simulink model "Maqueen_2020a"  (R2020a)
settings: Solver=VariableStepAuto  StartTime=0.0  StopTime=2  RelTol=1e-3
model workspace: external: MAT-File (data not in the file)
undefined symbols (not defined in the file or in its folder): deg, kg, m, mm, N, rad, s, smiData, X, Y, Z
libraries: sm_lib x459, fl_lib x12, nesl_utility x10
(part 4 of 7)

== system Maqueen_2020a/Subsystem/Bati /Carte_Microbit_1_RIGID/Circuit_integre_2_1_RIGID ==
  ReferenceFrame : sm_lib/Frames and Transforms/Reference Frame
  Solid : sm_lib/Body Elements/File Solid  ExtGeomFileName=Circuit integre 2_Defaut_sldprt.STL  UnitType=Custom  ExtGeomFileUnits=mm  StepReaderType=HEX  ExportConvexHullGeometry=off  InertiaType=Custom  Mass=smiData.Solid(13).mass  MassUnits=kg  CenterOfMass=smiData.Solid(13).CoM  CenterOfMassUnits=mm  MomentsOfInertia=smiData.Solid(13).MoI  MomentsOfInertiaUnits=kg*mm^2  ProductsOfInertia=smiData.Solid(13).PoI  ProductsOfInertiaUnits=kg*mm^2  BasedOnType=Density  Density=1000  DensityUnits=kg/m^3  DoExposeReferenceFrame=on  SerializedFrames=<Frames/>  GraphicType=FromGeometry  MarkerShape=Sphere  MarkerSize=10  GraphicVisPropType=SimpleVisualProperties  GraphicDiffuseColor=smiData.Solid(13).color  GraphicSpecularColor=[0.5 0.5 0.5 1.0]  GraphicAmbientColor=[0.15 0.15 0.15 1.0]  GraphicEmissiveColor=[0.0 0.0 0.0 1.0]  GraphicShininess=75  GraphicOpacity=smiData.Solid(13).opacity
  F : PMIOPort  Side=Left
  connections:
  ReferenceFrame/RConn1 -- Solid/RConn1 -- F/RConn1

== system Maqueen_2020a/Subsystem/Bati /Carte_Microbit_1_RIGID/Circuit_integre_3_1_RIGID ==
  ReferenceFrame : sm_lib/Frames and Transforms/Reference Frame
  Solid : sm_lib/Body Elements/File Solid  ExtGeomFileName=Circuit integre 3_Defaut_sldprt.STL  UnitType=Custom  ExtGeomFileUnits=mm  StepReaderType=HEX  ExportConvexHullGeometry=off  InertiaType=Custom  Mass=smiData.Solid(17).mass  MassUnits=kg  CenterOfMass=smiData.Solid(17).CoM  CenterOfMassUnits=mm  MomentsOfInertia=smiData.Solid(17).MoI  MomentsOfInertiaUnits=kg*mm^2  ProductsOfInertia=smiData.Solid(17).PoI  ProductsOfInertiaUnits=kg*mm^2  BasedOnType=Density  Density=1000  DensityUnits=kg/m^3  DoExposeReferenceFrame=on  SerializedFrames=<Frames/>  GraphicType=FromGeometry  MarkerShape=Sphere  MarkerSize=10  GraphicVisPropType=SimpleVisualProperties  GraphicDiffuseColor=smiData.Solid(17).color  GraphicSpecularColor=[0.5 0.5 0.5 1.0]  GraphicAmbientColor=[0.15 0.15 0.15 1.0]  GraphicEmissiveColor=[0.0 0.0 0.0 1.0]  GraphicShininess=75  GraphicOpacity=smiData.Solid(17).opacity
  F : PMIOPort  Side=Left
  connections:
  ReferenceFrame/RConn1 -- Solid/RConn1 -- F/RConn1

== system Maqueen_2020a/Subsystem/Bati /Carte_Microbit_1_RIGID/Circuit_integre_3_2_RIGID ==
  ReferenceFrame : sm_lib/Frames and Transforms/Reference Frame
  Solid : sm_lib/Body Elements/File Solid  ExtGeomFileName=Circuit integre 3_Defaut_sldprt.STL  UnitType=Custom  ExtGeomFileUnits=mm  StepReaderType=HEX  ExportConvexHullGeometry=off  InertiaType=Custom  Mass=smiData.Solid(17).mass  MassUnits=kg  CenterOfMass=smiData.Solid(17).CoM  CenterOfMassUnits=mm  MomentsOfInertia=smiData.Solid(17).MoI  MomentsOfInertiaUnits=kg*mm^2  ProductsOfInertia=smiData.Solid(17).PoI  ProductsOfInertiaUnits=kg*mm^2  BasedOnType=Density  Density=1000  DensityUnits=kg/m^3  DoExposeReferenceFrame=on  SerializedFrames=<Frames/>  GraphicType=FromGeometry  MarkerShape=Sphere  MarkerSize=10  GraphicVisPropType=SimpleVisualProperties  GraphicDiffuseColor=smiData.Solid(17).color  GraphicSpecularColor=[0.5 0.5 0.5 1.0]  GraphicAmbientColor=[0.15 0.15 0.15 1.0]  GraphicEmissiveColor=[0.0 0.0 0.0 1.0]  GraphicShininess=75  GraphicOpacity=smiData.Solid(17).opacity
  F : PMIOPort  Side=Left
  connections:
  ReferenceFrame/RConn1 -- Solid/RConn1 -- F/RConn1

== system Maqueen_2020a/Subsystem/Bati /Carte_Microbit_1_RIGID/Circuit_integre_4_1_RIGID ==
  ReferenceFrame : sm_lib/Frames and Transforms/Reference Frame
  Solid : sm_lib/Body Elements/File Solid  ExtGeomFileName=Circuit integre 4_Defaut_sldprt.STL  UnitType=Custom  ExtGeomFileUnits=mm  StepReaderType=HEX  ExportConvexHullGeometry=off  InertiaType=Custom  Mass=smiData.Solid(12).mass  MassUnits=kg  CenterOfMass=smiData.Solid(12).CoM  CenterOfMassUnits=mm  MomentsOfInertia=smiData.Solid(12).MoI  MomentsOfInertiaUnits=kg*mm^2  ProductsOfInertia=smiData.Solid(12).PoI  ProductsOfInertiaUnits=kg*mm^2  BasedOnType=Density  Density=1000  DensityUnits=kg/m^3  DoExposeReferenceFrame=on  SerializedFrames=<Frames/>  GraphicType=FromGeometry  MarkerShape=Sphere  MarkerSize=10  GraphicVisPropType=SimpleVisualProperties  GraphicDiffuseColor=smiData.Solid(12).color  GraphicSpecularColor=[0.5 0.5 0.5 1.0]  GraphicAmbientColor=[0.15 0.15 0.15 1.0]  GraphicEmissiveColor=[0.0 0.0 0.0 1.0]  GraphicShininess=75  GraphicOpacity=smiData.Solid(12).opacity
  F : PMIOPort  Side=Left
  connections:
  ReferenceFrame/RConn1 -- Solid/RConn1 -- F/RConn1

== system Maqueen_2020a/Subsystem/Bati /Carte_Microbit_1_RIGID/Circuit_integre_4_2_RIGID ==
  ReferenceFrame : sm_lib/Frames and Transforms/Reference Frame
  Solid : sm_lib/Body Elements/File Solid  ExtGeomFileName=Circuit integre 4_Defaut_sldprt.STL  UnitType=Custom  ExtGeomFileUnits=mm  StepReaderType=HEX  ExportConvexHullGeometry=off  InertiaType=Custom  Mass=smiData.Solid(12).mass  MassUnits=kg  CenterOfMass=smiData.Solid(12).CoM  CenterOfMassUnits=mm  MomentsOfInertia=smiData.Solid(12).MoI  MomentsOfInertiaUnits=kg*mm^2  ProductsOfInertia=smiData.Solid(12).PoI  ProductsOfInertiaUnits=kg*mm^2  BasedOnType=Density  Density=1000  DensityUnits=kg/m^3  DoExposeReferenceFrame=on  SerializedFrames=<Frames/>  GraphicType=FromGeometry  MarkerShape=Sphere  MarkerSize=10  GraphicVisPropType=SimpleVisualProperties  GraphicDiffuseColor=smiData.Solid(12).color  GraphicSpecularColor=[0.5 0.5 0.5 1.0]  GraphicAmbientColor=[0.15 0.15 0.15 1.0]  GraphicEmissiveColor=[0.0 0.0 0.0 1.0]  GraphicShininess=75  GraphicOpacity=smiData.Solid(12).opacity
  F : PMIOPort  Side=Left
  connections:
  ReferenceFrame/RConn1 -- Solid/RConn1 -- F/RConn1

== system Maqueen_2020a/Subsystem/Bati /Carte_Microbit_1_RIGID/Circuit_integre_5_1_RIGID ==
  ReferenceFrame : sm_lib/Frames and Transforms/Reference Frame
  Solid : sm_lib/Body Elements/File Solid  ExtGeomFileName=Circuit integre 5_Defaut_sldprt.STL  UnitType=Custom  ExtGeomFileUnits=mm  StepReaderType=HEX  ExportConvexHullGeometry=off  InertiaType=Custom  Mass=smiData.Solid(14).mass  MassUnits=kg  CenterOfMass=smiData.Solid(14).CoM  CenterOfMassUnits=mm  MomentsOfInertia=smiData.Solid(14).MoI  MomentsOfInertiaUnits=kg*mm^2  ProductsOfInertia=smiData.Solid(14).PoI  ProductsOfInertiaUnits=kg*mm^2  BasedOnType=Density  Density=1000  DensityUnits=kg/m^3  DoExposeReferenceFrame=on  SerializedFrames=<Frames/>  GraphicType=FromGeometry  MarkerShape=Sphere  MarkerSize=10  GraphicVisPropType=SimpleVisualProperties  GraphicDiffuseColor=smiData.Solid(14).color  GraphicSpecularColor=[0.5 0.5 0.5 1.0]  GraphicAmbientColor=[0.15 0.15 0.15 1.0]  GraphicEmissiveColor=[0.0 0.0 0.0 1.0]  GraphicShininess=75  GraphicOpacity=smiData.Solid(14).opacity
  F : PMIOPort  Side=Left
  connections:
  ReferenceFrame/RConn1 -- Solid/RConn1 -- F/RConn1

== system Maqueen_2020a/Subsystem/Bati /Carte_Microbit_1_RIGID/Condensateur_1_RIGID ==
  ReferenceFrame : sm_lib/Frames and Transforms/Reference Frame
  Solid : sm_lib/Body Elements/File Solid  ExtGeomFileName=Condensateur_Defaut_sldprt.STL  UnitType=Custom  ExtGeomFileUnits=mm  StepReaderType=HEX  ExportConvexHullGeometry=off  InertiaType=Custom  Mass=smiData.Solid(9).mass  MassUnits=kg  CenterOfMass=smiData.Solid(9).CoM  CenterOfMassUnits=mm  MomentsOfInertia=smiData.Solid(9).MoI  MomentsOfInertiaUnits=kg*mm^2  ProductsOfInertia=smiData.Solid(9).PoI  ProductsOfInertiaUnits=kg*mm^2  BasedOnType=Density  Density=1000  DensityUnits=kg/m^3  DoExposeReferenceFrame=on  SerializedFrames=<Frames/>  GraphicType=FromGeometry  MarkerShape=Sphere  MarkerSize=10  GraphicVisPropType=SimpleVisualProperties  GraphicDiffuseColor=smiData.Solid(9).color  GraphicSpecularColor=[0.5 0.5 0.5 1.0]  GraphicAmbientColor=[0.15 0.15 0.15 1.0]  GraphicEmissiveColor=[0.0 0.0 0.0 1.0]  GraphicShininess=75  GraphicOpacity=smiData.Solid(9).opacity
  F : PMIOPort  Side=Left
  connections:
  ReferenceFrame/RConn1 -- Solid/RConn1 -- F/RConn1

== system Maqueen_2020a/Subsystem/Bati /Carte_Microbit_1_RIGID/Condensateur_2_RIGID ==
  ReferenceFrame : sm_lib/Frames and Transforms/Reference Frame
  Solid : sm_lib/Body Elements/File Solid  ExtGeomFileName=Condensateur_Defaut_sldprt.STL  UnitType=Custom  ExtGeomFileUnits=mm  StepReaderType=HEX  ExportConvexHullGeometry=off  InertiaType=Custom  Mass=smiData.Solid(9).mass  MassUnits=kg  CenterOfMass=smiData.Solid(9).CoM  CenterOfMassUnits=mm  MomentsOfInertia=smiData.Solid(9).MoI  MomentsOfInertiaUnits=kg*mm^2  ProductsOfInertia=smiData.Solid(9).PoI  ProductsOfInertiaUnits=kg*mm^2  BasedOnType=Density  Density=1000  DensityUnits=kg/m^3  DoExposeReferenceFrame=on  SerializedFrames=<Frames/>  GraphicType=FromGeometry  MarkerShape=Sphere  MarkerSize=10  GraphicVisPropType=SimpleVisualProperties  GraphicDiffuseColor=smiData.Solid(9).color  GraphicSpecularColor=[0.5 0.5 0.5 1.0]  GraphicAmbientColor=[0.15 0.15 0.15 1.0]  GraphicEmissiveColor=[0.0 0.0 0.0 1.0]  GraphicShininess=75  GraphicOpacity=smiData.Solid(9).opacity
  F : PMIOPort  Side=Left
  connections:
  ReferenceFrame/RConn1 -- Solid/RConn1 -- F/RConn1

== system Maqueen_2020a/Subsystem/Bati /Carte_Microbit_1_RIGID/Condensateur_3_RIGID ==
  ReferenceFrame : sm_lib/Frames and Transforms/Reference Frame
  Solid : sm_lib/Body Elements/File Solid  ExtGeomFileName=Condensateur_Defaut_sldprt.STL  UnitType=Custom  ExtGeomFileUnits=mm  StepReaderType=HEX  ExportConvexHullGeometry=off  InertiaType=Custom  Mass=smiData.Solid(9).mass  MassUnits=kg  CenterOfMass=smiData.Solid(9).CoM  CenterOfMassUnits=mm  MomentsOfInertia=smiData.Solid(9).MoI  MomentsOfInertiaUnits=kg*mm^2  ProductsOfInertia=smiData.Solid(9).PoI  ProductsOfInertiaUnits=kg*mm^2  BasedOnType=Density  Density=1000  DensityUnits=kg/m^3  DoExposeReferenceFrame=on  SerializedFrames=<Frames/>  GraphicType=FromGeometry  MarkerShape=Sphere  MarkerSize=10  GraphicVisPropType=SimpleVisualProperties  GraphicDiffuseColor=smiData.Solid(9).color  GraphicSpecularColor=[0.5 0.5 0.5 1.0]  GraphicAmbientColor=[0.15 0.15 0.15 1.0]  GraphicEmissiveColor=[0.0 0.0 0.0 1.0]  GraphicShininess=75  GraphicOpacity=smiData.Solid(9).opacity
  F : PMIOPort  Side=Left
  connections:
  ReferenceFrame/RConn1 -- Solid/RConn1 -- F/RConn1

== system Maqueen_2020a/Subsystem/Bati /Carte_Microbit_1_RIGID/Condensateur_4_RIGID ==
  ReferenceFrame : sm_lib/Frames and Transforms/Reference Frame
  Solid : sm_lib/Body Elements/File Solid  ExtGeomFileName=Condensateur_Defaut_sldprt.STL  UnitType=Custom  ExtGeomFileUnits=mm  StepReaderType=HEX  ExportConvexHullGeometry=off  InertiaType=Custom  Mass=smiData.Solid(9).mass  MassUnits=kg  CenterOfMass=smiData.Solid(9).CoM  CenterOfMassUnits=mm  MomentsOfInertia=smiData.Solid(9).MoI  MomentsOfInertiaUnits=kg*mm^2  ProductsOfInertia=smiData.Solid(9).PoI  ProductsOfInertiaUnits=kg*mm^2  BasedOnType=Density  Density=1000  DensityUnits=kg/m^3  DoExposeReferenceFrame=on  SerializedFrames=<Frames/>  GraphicType=FromGeometry  MarkerShape=Sphere  MarkerSize=10  GraphicVisPropType=SimpleVisualProperties  GraphicDiffuseColor=smiData.Solid(9).color  GraphicSpecularColor=[0.5 0.5 0.5 1.0]  GraphicAmbientColor=[0.15 0.15 0.15 1.0]  GraphicEmissiveColor=[0.0 0.0 0.0 1.0]  GraphicShininess=75  GraphicOpacity=smiData.Solid(9).opacity
  F : PMIOPort  Side=Left
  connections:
  ReferenceFrame/RConn1 -- Solid/RConn1 -- F/RConn1

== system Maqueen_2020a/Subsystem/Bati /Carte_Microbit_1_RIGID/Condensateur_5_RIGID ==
  ReferenceFrame : sm_lib/Frames and Transforms/Reference Frame
  Solid : sm_lib/Body Elements/File Solid  ExtGeomFileName=Condensateur_Defaut_sldprt.STL  UnitType=Custom  ExtGeomFileUnits=mm  StepReaderType=HEX  ExportConvexHullGeometry=off  InertiaType=Custom  Mass=smiData.Solid(9).mass  MassUnits=kg  CenterOfMass=smiData.Solid(9).CoM  CenterOfMassUnits=mm  MomentsOfInertia=smiData.Solid(9).MoI  MomentsOfInertiaUnits=kg*mm^2  ProductsOfInertia=smiData.Solid(9).PoI  ProductsOfInertiaUnits=kg*mm^2  BasedOnType=Density  Density=1000  DensityUnits=kg/m^3  DoExposeReferenceFrame=on  SerializedFrames=<Frames/>  GraphicType=FromGeometry  MarkerShape=Sphere  MarkerSize=10  GraphicVisPropType=SimpleVisualProperties  GraphicDiffuseColor=smiData.Solid(9).color  GraphicSpecularColor=[0.5 0.5 0.5 1.0]  GraphicAmbientColor=[0.15 0.15 0.15 1.0]  GraphicEmissiveColor=[0.0 0.0 0.0 1.0]  GraphicShininess=75  GraphicOpacity=smiData.Solid(9).opacity
  F : PMIOPort  Side=Left
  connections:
  ReferenceFrame/RConn1 -- Solid/RConn1 -- F/RConn1

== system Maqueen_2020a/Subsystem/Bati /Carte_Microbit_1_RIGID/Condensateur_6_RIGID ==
  ReferenceFrame : sm_lib/Frames and Transforms/Reference Frame
  Solid : sm_lib/Body Elements/File Solid  ExtGeomFileName=Condensateur_Defaut_sldprt.STL  UnitType=Custom  ExtGeomFileUnits=mm  StepReaderType=HEX  ExportConvexHullGeometry=off  InertiaType=Custom  Mass=smiData.Solid(9).mass  MassUnits=kg  CenterOfMass=smiData.Solid(9).CoM  CenterOfMassUnits=mm  MomentsOfInertia=smiData.Solid(9).MoI  MomentsOfInertiaUnits=kg*mm^2  ProductsOfInertia=smiData.Solid(9).PoI  ProductsOfInertiaUnits=kg*mm^2  BasedOnType=Density  Density=1000  DensityUnits=kg/m^3  DoExposeReferenceFrame=on  SerializedFrames=<Frames/>  GraphicType=FromGeometry  MarkerShape=Sphere  MarkerSize=10  GraphicVisPropType=SimpleVisualProperties  GraphicDiffuseColor=smiData.Solid(9).color  GraphicSpecularColor=[0.5 0.5 0.5 1.0]  GraphicAmbientColor=[0.15 0.15 0.15 1.0]  GraphicEmissiveColor=[0.0 0.0 0.0 1.0]  GraphicShininess=75  GraphicOpacity=smiData.Solid(9).opacity
  F : PMIOPort  Side=Left
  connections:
  ReferenceFrame/RConn1 -- Solid/RConn1 -- F/RConn1

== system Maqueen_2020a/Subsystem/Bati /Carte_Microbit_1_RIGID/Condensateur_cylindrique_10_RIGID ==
  ReferenceFrame : sm_lib/Frames and Transforms/Reference Frame
  Solid : sm_lib/Body Elements/File Solid  ExtGeomFileName=Condensateur cylindrique_Defaut_sldprt.STL  UnitType=Custom  ExtGeomFileUnits=mm  StepReaderType=HEX  ExportConvexHullGeometry=off  InertiaType=Custom  Mass=smiData.Solid(8).mass  MassUnits=kg  CenterOfMass=smiData.Solid(8).CoM  CenterOfMassUnits=mm  MomentsOfInertia=smiData.Solid(8).MoI  MomentsOfInertiaUnits=kg*mm^2  ProductsOfInertia=smiData.Solid(8).PoI  ProductsOfInertiaUnits=kg*mm^2  BasedOnType=Density  Density=1000  DensityUnits=kg/m^3  DoExposeReferenceFrame=on  SerializedFrames=<Frames/>  GraphicType=FromGeometry  MarkerShape=Sphere  MarkerSize=10  GraphicVisPropType=SimpleVisualProperties  GraphicDiffuseColor=smiData.Solid(8).color  GraphicSpecularColor=[0.5 0.5 0.5 1.0]  GraphicAmbientColor=[0.15 0.15 0.15 1.0]  GraphicEmissiveColor=[0.0 0.0 0.0 1.0]  GraphicShininess=75  GraphicOpacity=smiData.Solid(8).opacity
  F : PMIOPort  Side=Left
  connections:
  ReferenceFrame/RConn1 -- Solid/RConn1 -- F/RConn1

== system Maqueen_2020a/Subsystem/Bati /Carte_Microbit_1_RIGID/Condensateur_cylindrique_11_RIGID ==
  ReferenceFrame : sm_lib/Frames and Transforms/Reference Frame
  Solid : sm_lib/Body Elements/File Solid  ExtGeomFileName=Condensateur cylindrique_Defaut_sldprt.STL  UnitType=Custom  ExtGeomFileUnits=mm  StepReaderType=HEX  ExportConvexHullGeometry=off  InertiaType=Custom  Mass=smiData.Solid(8).mass  MassUnits=kg  CenterOfMass=smiData.Solid(8).CoM  CenterOfMassUnits=mm  MomentsOfInertia=smiData.Solid(8).MoI  MomentsOfInertiaUnits=kg*mm^2  ProductsOfInertia=smiData.Solid(8).PoI  ProductsOfInertiaUnits=kg*mm^2  BasedOnType=Density  Density=1000  DensityUnits=kg/m^3  DoExposeReferenceFrame=on  SerializedFrames=<Frames/>  GraphicType=FromGeometry  MarkerShape=Sphere  MarkerSize=10  GraphicVisPropType=SimpleVisualProperties  GraphicDiffuseColor=smiData.Solid(8).color  GraphicSpecularColor=[0.5 0.5 0.5 1.0]  GraphicAmbientColor=[0.15 0.15 0.15 1.0]  GraphicEmissiveColor=[0.0 0.0 0.0 1.0]  GraphicShininess=75  GraphicOpacity=smiData.Solid(8).opacity
  F : PMIOPort  Side=Left
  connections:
  ReferenceFrame/RConn1 -- Solid/RConn1 -- F/RConn1

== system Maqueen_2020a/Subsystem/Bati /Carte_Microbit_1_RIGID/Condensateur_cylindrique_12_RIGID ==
  ReferenceFrame : sm_lib/Frames and Transforms/Reference Frame
  Solid : sm_lib/Body Elements/File Solid  ExtGeomFileName=Condensateur cylindrique_Defaut_sldprt.STL  UnitType=Custom  ExtGeomFileUnits=mm  StepReaderType=HEX  ExportConvexHullGeometry=off  InertiaType=Custom  Mass=smiData.Solid(8).mass  MassUnits=kg  CenterOfMass=smiData.Solid(8).CoM  CenterOfMassUnits=mm  MomentsOfInertia=smiData.Solid(8).MoI  MomentsOfInertiaUnits=kg*mm^2  ProductsOfInertia=smiData.Solid(8).PoI  ProductsOfInertiaUnits=kg*mm^2  BasedOnType=Density  Density=1000  DensityUnits=kg/m^3  DoExposeReferenceFrame=on  SerializedFrames=<Frames/>  GraphicType=FromGeometry  MarkerShape=Sphere  MarkerSize=10  GraphicVisPropType=SimpleVisualProperties  GraphicDiffuseColor=smiData.Solid(8).color  GraphicSpecularColor=[0.5 0.5 0.5 1.0]  GraphicAmbientColor=[0.15 0.15 0.15 1.0]  GraphicEmissiveColor=[0.0 0.0 0.0 1.0]  GraphicShininess=75  GraphicOpacity=smiData.Solid(8).opacity
  F : PMIOPort  Side=Left
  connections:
  ReferenceFrame/RConn1 -- Solid/RConn1 -- F/RConn1

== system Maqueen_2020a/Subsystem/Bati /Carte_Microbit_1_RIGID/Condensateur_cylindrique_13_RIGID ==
  ReferenceFrame : sm_lib/Frames and Transforms/Reference Frame
  Solid : sm_lib/Body Elements/File Solid  ExtGeomFileName=Condensateur cylindrique_Defaut_sldprt.STL  UnitType=Custom  ExtGeomFileUnits=mm  StepReaderType=HEX  ExportConvexHullGeometry=off  InertiaType=Custom  Mass=smiData.Solid(8).mass  MassUnits=kg  CenterOfMass=smiData.Solid(8).CoM  CenterOfMassUnits=mm  MomentsOfInertia=smiData.Solid(8).MoI  MomentsOfInertiaUnits=kg*mm^2  ProductsOfInertia=smiData.Solid(8).PoI  ProductsOfInertiaUnits=kg*mm^2  BasedOnType=Density  Density=1000  DensityUnits=kg/m^3  DoExposeReferenceFrame=on  SerializedFrames=<Frames/>  GraphicType=FromGeometry  MarkerShape=Sphere  MarkerSize=10  GraphicVisPropType=SimpleVisualProperties  GraphicDiffuseColor=smiData.Solid(8).color  GraphicSpecularColor=[0.5 0.5 0.5 1.0]  GraphicAmbientColor=[0.15 0.15 0.15 1.0]  GraphicEmissiveColor=[0.0 0.0 0.0 1.0]  GraphicShininess=75  GraphicOpacity=smiData.Solid(8).opacity
  F : PMIOPort  Side=Left
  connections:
  ReferenceFrame/RConn1 -- Solid/RConn1 -- F/RConn1

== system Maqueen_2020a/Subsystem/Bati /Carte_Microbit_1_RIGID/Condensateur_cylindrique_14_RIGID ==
  ReferenceFrame : sm_lib/Frames and Transforms/Reference Frame
  Solid : sm_lib/Body Elements/File Solid  ExtGeomFileName=Condensateur cylindrique_Defaut_sldprt.STL  UnitType=Custom  ExtGeomFileUnits=mm  StepReaderType=HEX  ExportConvexHullGeometry=off  InertiaType=Custom  Mass=smiData.Solid(8).mass  MassUnits=kg  CenterOfMass=smiData.Solid(8).CoM  CenterOfMassUnits=mm  MomentsOfInertia=smiData.Solid(8).MoI  MomentsOfInertiaUnits=kg*mm^2  ProductsOfInertia=smiData.Solid(8).PoI  ProductsOfInertiaUnits=kg*mm^2  BasedOnType=Density  Density=1000  DensityUnits=kg/m^3  DoExposeReferenceFrame=on  SerializedFrames=<Frames/>  GraphicType=FromGeometry  MarkerShape=Sphere  MarkerSize=10  GraphicVisPropType=SimpleVisualProperties  GraphicDiffuseColor=smiData.Solid(8).color  GraphicSpecularColor=[0.5 0.5 0.5 1.0]  GraphicAmbientColor=[0.15 0.15 0.15 1.0]  GraphicEmissiveColor=[0.0 0.0 0.0 1.0]  GraphicShininess=75  GraphicOpacity=smiData.Solid(8).opacity
  F : PMIOPort  Side=Left
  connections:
  ReferenceFrame/RConn1 -- Solid/RConn1 -- F/RConn1

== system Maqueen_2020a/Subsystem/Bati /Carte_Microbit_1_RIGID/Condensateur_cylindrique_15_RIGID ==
  ReferenceFrame : sm_lib/Frames and Transforms/Reference Frame
  Solid : sm_lib/Body Elements/File Solid  ExtGeomFileName=Condensateur cylindrique_Defaut_sldprt.STL  UnitType=Custom  ExtGeomFileUnits=mm  StepReaderType=HEX  ExportConvexHullGeometry=off  InertiaType=Custom  Mass=smiData.Solid(8).mass  MassUnits=kg  CenterOfMass=smiData.Solid(8).CoM  CenterOfMassUnits=mm  MomentsOfInertia=smiData.Solid(8).MoI  MomentsOfInertiaUnits=kg*mm^2  ProductsOfInertia=smiData.Solid(8).PoI  ProductsOfInertiaUnits=kg*mm^2  BasedOnType=Density  Density=1000  DensityUnits=kg/m^3  DoExposeReferenceFrame=on  SerializedFrames=<Frames/>  GraphicType=FromGeometry  MarkerShape=Sphere  MarkerSize=10  GraphicVisPropType=SimpleVisualProperties  GraphicDiffuseColor=smiData.Solid(8).color  GraphicSpecularColor=[0.5 0.5 0.5 1.0]  GraphicAmbientColor=[0.15 0.15 0.15 1.0]  GraphicEmissiveColor=[0.0 0.0 0.0 1.0]  GraphicShininess=75  GraphicOpacity=smiData.Solid(8).opacity
  F : PMIOPort  Side=Left
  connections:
  ReferenceFrame/RConn1 -- Solid/RConn1 -- F/RConn1

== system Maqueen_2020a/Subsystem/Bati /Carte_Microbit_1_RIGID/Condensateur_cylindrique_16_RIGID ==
  ReferenceFrame : sm_lib/Frames and Transforms/Reference Frame
  Solid : sm_lib/Body Elements/File Solid  ExtGeomFileName=Condensateur cylindrique_Defaut_sldprt.STL  UnitType=Custom  ExtGeomFileUnits=mm  StepReaderType=HEX  ExportConvexHullGeometry=off  InertiaType=Custom  Mass=smiData.Solid(8).mass  MassUnits=kg  CenterOfMass=smiData.Solid(8).CoM  CenterOfMassUnits=mm  MomentsOfInertia=smiData.Solid(8).MoI  MomentsOfInertiaUnits=kg*mm^2  ProductsOfInertia=smiData.Solid(8).PoI  ProductsOfInertiaUnits=kg*mm^2  BasedOnType=Density  Density=1000  DensityUnits=kg/m^3  DoExposeReferenceFrame=on  SerializedFrames=<Frames/>  GraphicType=FromGeometry  MarkerShape=Sphere  MarkerSize=10  GraphicVisPropType=SimpleVisualProperties  GraphicDiffuseColor=smiData.Solid(8).color  GraphicSpecularColor=[0.5 0.5 0.5 1.0]  GraphicAmbientColor=[0.15 0.15 0.15 1.0]  GraphicEmissiveColor=[0.0 0.0 0.0 1.0]  GraphicShininess=75  GraphicOpacity=smiData.Solid(8).opacity
  F : PMIOPort  Side=Left
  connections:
  ReferenceFrame/RConn1 -- Solid/RConn1 -- F/RConn1

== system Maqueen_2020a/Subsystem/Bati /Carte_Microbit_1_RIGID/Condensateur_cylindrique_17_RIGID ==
  ReferenceFrame : sm_lib/Frames and Transforms/Reference Frame
  Solid : sm_lib/Body Elements/File Solid  ExtGeomFileName=Condensateur cylindrique_Defaut_sldprt.STL  UnitType=Custom  ExtGeomFileUnits=mm  StepReaderType=HEX  ExportConvexHullGeometry=off  InertiaType=Custom  Mass=smiData.Solid(8).mass  MassUnits=kg  CenterOfMass=smiData.Solid(8).CoM  CenterOfMassUnits=mm  MomentsOfInertia=smiData.Solid(8).MoI  MomentsOfInertiaUnits=kg*mm^2  ProductsOfInertia=smiData.Solid(8).PoI  ProductsOfInertiaUnits=kg*mm^2  BasedOnType=Density  Density=1000  DensityUnits=kg/m^3  DoExposeReferenceFrame=on  SerializedFrames=<Frames/>  GraphicType=FromGeometry  MarkerShape=Sphere  MarkerSize=10  GraphicVisPropType=SimpleVisualProperties  GraphicDiffuseColor=smiData.Solid(8).color  GraphicSpecularColor=[0.5 0.5 0.5 1.0]  GraphicAmbientColor=[0.15 0.15 0.15 1.0]  GraphicEmissiveColor=[0.0 0.0 0.0 1.0]  GraphicShininess=75  GraphicOpacity=smiData.Solid(8).opacity
  F : PMIOPort  Side=Left
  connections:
  ReferenceFrame/RConn1 -- Solid/RConn1 -- F/RConn1

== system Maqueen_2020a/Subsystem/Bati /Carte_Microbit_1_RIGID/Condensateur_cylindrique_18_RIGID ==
  ReferenceFrame : sm_lib/Frames and Transforms/Reference Frame
  Solid : sm_lib/Body Elements/File Solid  ExtGeomFileName=Condensateur cylindrique_Defaut_sldprt.STL  UnitType=Custom  ExtGeomFileUnits=mm  StepReaderType=HEX  ExportConvexHullGeometry=off  InertiaType=Custom  Mass=smiData.Solid(8).mass  MassUnits=kg  CenterOfMass=smiData.Solid(8).CoM  CenterOfMassUnits=mm  MomentsOfInertia=smiData.Solid(8).MoI  MomentsOfInertiaUnits=kg*mm^2  ProductsOfInertia=smiData.Solid(8).PoI  ProductsOfInertiaUnits=kg*mm^2  BasedOnType=Density  Density=1000  DensityUnits=kg/m^3  DoExposeReferenceFrame=on  SerializedFrames=<Frames/>  GraphicType=FromGeometry  MarkerShape=Sphere  MarkerSize=10  GraphicVisPropType=SimpleVisualProperties  GraphicDiffuseColor=smiData.Solid(8).color  GraphicSpecularColor=[0.5 0.5 0.5 1.0]  GraphicAmbientColor=[0.15 0.15 0.15 1.0]  GraphicEmissiveColor=[0.0 0.0 0.0 1.0]  GraphicShininess=75  GraphicOpacity=smiData.Solid(8).opacity
  F : PMIOPort  Side=Left
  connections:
  ReferenceFrame/RConn1 -- Solid/RConn1 -- F/RConn1

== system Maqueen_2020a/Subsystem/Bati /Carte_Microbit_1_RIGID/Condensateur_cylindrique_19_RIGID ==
  ReferenceFrame : sm_lib/Frames and Transforms/Reference Frame
  Solid : sm_lib/Body Elements/File Solid  ExtGeomFileName=Condensateur cylindrique_Defaut_sldprt.STL  UnitType=Custom  ExtGeomFileUnits=mm  StepReaderType=HEX  ExportConvexHullGeometry=off  InertiaType=Custom  Mass=smiData.Solid(8).mass  MassUnits=kg  CenterOfMass=smiData.Solid(8).CoM  CenterOfMassUnits=mm  MomentsOfInertia=smiData.Solid(8).MoI  MomentsOfInertiaUnits=kg*mm^2  ProductsOfInertia=smiData.Solid(8).PoI  ProductsOfInertiaUnits=kg*mm^2  BasedOnType=Density  Density=1000  DensityUnits=kg/m^3  DoExposeReferenceFrame=on  SerializedFrames=<Frames/>  GraphicType=FromGeometry  MarkerShape=Sphere  MarkerSize=10  GraphicVisPropType=SimpleVisualProperties  GraphicDiffuseColor=smiData.Solid(8).color  GraphicSpecularColor=[0.5 0.5 0.5 1.0]  GraphicAmbientColor=[0.15 0.15 0.15 1.0]  GraphicEmissiveColor=[0.0 0.0 0.0 1.0]  GraphicShininess=75  GraphicOpacity=smiData.Solid(8).opacity
  F : PMIOPort  Side=Left
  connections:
  ReferenceFrame/RConn1 -- Solid/RConn1 -- F/RConn1

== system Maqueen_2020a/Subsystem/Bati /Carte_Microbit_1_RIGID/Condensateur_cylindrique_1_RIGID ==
  ReferenceFrame : sm_lib/Frames and Transforms/Reference Frame
  Solid : sm_lib/Body Elements/File Solid  ExtGeomFileName=Condensateur cylindrique_Defaut_sldprt.STL  UnitType=Custom  ExtGeomFileUnits=mm  StepReaderType=HEX  ExportConvexHullGeometry=off  InertiaType=Custom  Mass=smiData.Solid(8).mass  MassUnits=kg  CenterOfMass=smiData.Solid(8).CoM  CenterOfMassUnits=mm  MomentsOfInertia=smiData.Solid(8).MoI  MomentsOfInertiaUnits=kg*mm^2  ProductsOfInertia=smiData.Solid(8).PoI  ProductsOfInertiaUnits=kg*mm^2  BasedOnType=Density  Density=1000  DensityUnits=kg/m^3  DoExposeReferenceFrame=on  SerializedFrames=<Frames/>  GraphicType=FromGeometry  MarkerShape=Sphere  MarkerSize=10  GraphicVisPropType=SimpleVisualProperties  GraphicDiffuseColor=smiData.Solid(8).color  GraphicSpecularColor=[0.5 0.5 0.5 1.0]  GraphicAmbientColor=[0.15 0.15 0.15 1.0]  GraphicEmissiveColor=[0.0 0.0 0.0 1.0]  GraphicShininess=75  GraphicOpacity=smiData.Solid(8).opacity
  F : PMIOPort  Side=Left
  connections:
  ReferenceFrame/RConn1 -- Solid/RConn1 -- F/RConn1

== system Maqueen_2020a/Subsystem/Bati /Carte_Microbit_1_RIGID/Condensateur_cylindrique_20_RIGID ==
  ReferenceFrame : sm_lib/Frames and Transforms/Reference Frame
  Solid : sm_lib/Body Elements/File Solid  ExtGeomFileName=Condensateur cylindrique_Defaut_sldprt.STL  UnitType=Custom  ExtGeomFileUnits=mm  StepReaderType=HEX  ExportConvexHullGeometry=off  InertiaType=Custom  Mass=smiData.Solid(8).mass  MassUnits=kg  CenterOfMass=smiData.Solid(8).CoM  CenterOfMassUnits=mm  MomentsOfInertia=smiData.Solid(8).MoI  MomentsOfInertiaUnits=kg*mm^2  ProductsOfInertia=smiData.Solid(8).PoI  ProductsOfInertiaUnits=kg*mm^2  BasedOnType=Density  Density=1000  DensityUnits=kg/m^3  DoExposeReferenceFrame=on  SerializedFrames=<Frames/>  GraphicType=FromGeometry  MarkerShape=Sphere  MarkerSize=10  GraphicVisPropType=SimpleVisualProperties  GraphicDiffuseColor=smiData.Solid(8).color  GraphicSpecularColor=[0.5 0.5 0.5 1.0]  GraphicAmbientColor=[0.15 0.15 0.15 1.0]  GraphicEmissiveColor=[0.0 0.0 0.0 1.0]  GraphicShininess=75  GraphicOpacity=smiData.Solid(8).opacity
  F : PMIOPort  Side=Left
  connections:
  ReferenceFrame/RConn1 -- Solid/RConn1 -- F/RConn1

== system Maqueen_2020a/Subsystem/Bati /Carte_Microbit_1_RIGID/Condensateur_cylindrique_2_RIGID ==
  ReferenceFrame : sm_lib/Frames and Transforms/Reference Frame
  Solid : sm_lib/Body Elements/File Solid  ExtGeomFileName=Condensateur cylindrique_Defaut_sldprt.STL  UnitType=Custom  ExtGeomFileUnits=mm  StepReaderType=HEX  ExportConvexHullGeometry=off  InertiaType=Custom  Mass=smiData.Solid(8).mass  MassUnits=kg  CenterOfMass=smiData.Solid(8).CoM  CenterOfMassUnits=mm  MomentsOfInertia=smiData.Solid(8).MoI  MomentsOfInertiaUnits=kg*mm^2  ProductsOfInertia=smiData.Solid(8).PoI  ProductsOfInertiaUnits=kg*mm^2  BasedOnType=Density  Density=1000  DensityUnits=kg/m^3  DoExposeReferenceFrame=on  SerializedFrames=<Frames/>  GraphicType=FromGeometry  MarkerShape=Sphere  MarkerSize=10  GraphicVisPropType=SimpleVisualProperties  GraphicDiffuseColor=smiData.Solid(8).color  GraphicSpecularColor=[0.5 0.5 0.5 1.0]  GraphicAmbientColor=[0.15 0.15 0.15 1.0]  GraphicEmissiveColor=[0.0 0.0 0.0 1.0]  GraphicShininess=75  GraphicOpacity=smiData.Solid(8).opacity
  F : PMIOPort  Side=Left
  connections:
  ReferenceFrame/RConn1 -- Solid/RConn1 -- F/RConn1

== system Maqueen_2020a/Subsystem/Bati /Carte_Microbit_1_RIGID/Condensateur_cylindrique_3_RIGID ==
  ReferenceFrame : sm_lib/Frames and Transforms/Reference Frame
  Solid : sm_lib/Body Elements/File Solid  ExtGeomFileName=Condensateur cylindrique_Defaut_sldprt.STL  UnitType=Custom  ExtGeomFileUnits=mm  StepReaderType=HEX  ExportConvexHullGeometry=off  InertiaType=Custom  Mass=smiData.Solid(8).mass  MassUnits=kg  CenterOfMass=smiData.Solid(8).CoM  CenterOfMassUnits=mm  MomentsOfInertia=smiData.Solid(8).MoI  MomentsOfInertiaUnits=kg*mm^2  ProductsOfInertia=smiData.Solid(8).PoI  ProductsOfInertiaUnits=kg*mm^2  BasedOnType=Density  Density=1000  DensityUnits=kg/m^3  DoExposeReferenceFrame=on  SerializedFrames=<Frames/>  GraphicType=FromGeometry  MarkerShape=Sphere  MarkerSize=10  GraphicVisPropType=SimpleVisualProperties  GraphicDiffuseColor=smiData.Solid(8).color  GraphicSpecularColor=[0.5 0.5 0.5 1.0]  GraphicAmbientColor=[0.15 0.15 0.15 1.0]  GraphicEmissiveColor=[0.0 0.0 0.0 1.0]  GraphicShininess=75  GraphicOpacity=smiData.Solid(8).opacity
  F : PMIOPort  Side=Left
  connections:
  ReferenceFrame/RConn1 -- Solid/RConn1 -- F/RConn1

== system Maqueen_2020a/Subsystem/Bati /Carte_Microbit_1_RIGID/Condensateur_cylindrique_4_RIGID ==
  ReferenceFrame : sm_lib/Frames and Transforms/Reference Frame
  Solid : sm_lib/Body Elements/File Solid  ExtGeomFileName=Condensateur cylindrique_Defaut_sldprt.STL  UnitType=Custom  ExtGeomFileUnits=mm  StepReaderType=HEX  ExportConvexHullGeometry=off  InertiaType=Custom  Mass=smiData.Solid(8).mass  MassUnits=kg  CenterOfMass=smiData.Solid(8).CoM  CenterOfMassUnits=mm  MomentsOfInertia=smiData.Solid(8).MoI  MomentsOfInertiaUnits=kg*mm^2  ProductsOfInertia=smiData.Solid(8).PoI  ProductsOfInertiaUnits=kg*mm^2  BasedOnType=Density  Density=1000  DensityUnits=kg/m^3  DoExposeReferenceFrame=on  SerializedFrames=<Frames/>  GraphicType=FromGeometry  MarkerShape=Sphere  MarkerSize=10  GraphicVisPropType=SimpleVisualProperties  GraphicDiffuseColor=smiData.Solid(8).color  GraphicSpecularColor=[0.5 0.5 0.5 1.0]  GraphicAmbientColor=[0.15 0.15 0.15 1.0]  GraphicEmissiveColor=[0.0 0.0 0.0 1.0]  GraphicShininess=75  GraphicOpacity=smiData.Solid(8).opacity
  F : PMIOPort  Side=Left
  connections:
  ReferenceFrame/RConn1 -- Solid/RConn1 -- F/RConn1

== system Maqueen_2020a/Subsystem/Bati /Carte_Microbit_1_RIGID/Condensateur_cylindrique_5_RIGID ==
  ReferenceFrame : sm_lib/Frames and Transforms/Reference Frame
  Solid : sm_lib/Body Elements/File Solid  ExtGeomFileName=Condensateur cylindrique_Defaut_sldprt.STL  UnitType=Custom  ExtGeomFileUnits=mm  StepReaderType=HEX  ExportConvexHullGeometry=off  InertiaType=Custom  Mass=smiData.Solid(8).mass  MassUnits=kg  CenterOfMass=smiData.Solid(8).CoM  CenterOfMassUnits=mm  MomentsOfInertia=smiData.Solid(8).MoI  MomentsOfInertiaUnits=kg*mm^2  ProductsOfInertia=smiData.Solid(8).PoI  ProductsOfInertiaUnits=kg*mm^2  BasedOnType=Density  Density=1000  DensityUnits=kg/m^3  DoExposeReferenceFrame=on  SerializedFrames=<Frames/>  GraphicType=FromGeometry  MarkerShape=Sphere  MarkerSize=10  GraphicVisPropType=SimpleVisualProperties  GraphicDiffuseColor=smiData.Solid(8).color  GraphicSpecularColor=[0.5 0.5 0.5 1.0]  GraphicAmbientColor=[0.15 0.15 0.15 1.0]  GraphicEmissiveColor=[0.0 0.0 0.0 1.0]  GraphicShininess=75  GraphicOpacity=smiData.Solid(8).opacity
  F : PMIOPort  Side=Left
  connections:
  ReferenceFrame/RConn1 -- Solid/RConn1 -- F/RConn1

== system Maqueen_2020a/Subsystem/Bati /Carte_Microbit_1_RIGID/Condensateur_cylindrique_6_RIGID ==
  ReferenceFrame : sm_lib/Frames and Transforms/Reference Frame
  Solid : sm_lib/Body Elements/File Solid  ExtGeomFileName=Condensateur cylindrique_Defaut_sldprt.STL  UnitType=Custom  ExtGeomFileUnits=mm  StepReaderType=HEX  ExportConvexHullGeometry=off  InertiaType=Custom  Mass=smiData.Solid(8).mass  MassUnits=kg  CenterOfMass=smiData.Solid(8).CoM  CenterOfMassUnits=mm  MomentsOfInertia=smiData.Solid(8).MoI  MomentsOfInertiaUnits=kg*mm^2  ProductsOfInertia=smiData.Solid(8).PoI  ProductsOfInertiaUnits=kg*mm^2  BasedOnType=Density  Density=1000  DensityUnits=kg/m^3  DoExposeReferenceFrame=on  SerializedFrames=<Frames/>  GraphicType=FromGeometry  MarkerShape=Sphere  MarkerSize=10  GraphicVisPropType=SimpleVisualProperties  GraphicDiffuseColor=smiData.Solid(8).color  GraphicSpecularColor=[0.5 0.5 0.5 1.0]  GraphicAmbientColor=[0.15 0.15 0.15 1.0]  GraphicEmissiveColor=[0.0 0.0 0.0 1.0]  GraphicShininess=75  GraphicOpacity=smiData.Solid(8).opacity
  F : PMIOPort  Side=Left
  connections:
  ReferenceFrame/RConn1 -- Solid/RConn1 -- F/RConn1

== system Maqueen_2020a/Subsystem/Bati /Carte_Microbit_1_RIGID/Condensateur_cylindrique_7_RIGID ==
  ReferenceFrame : sm_lib/Frames and Transforms/Reference Frame
  Solid : sm_lib/Body Elements/File Solid  ExtGeomFileName=Condensateur cylindrique_Defaut_sldprt.STL  UnitType=Custom  ExtGeomFileUnits=mm  StepReaderType=HEX  ExportConvexHullGeometry=off  InertiaType=Custom  Mass=smiData.Solid(8).mass  MassUnits=kg  CenterOfMass=smiData.Solid(8).CoM  CenterOfMassUnits=mm  MomentsOfInertia=smiData.Solid(8).MoI  MomentsOfInertiaUnits=kg*mm^2  ProductsOfInertia=smiData.Solid(8).PoI  ProductsOfInertiaUnits=kg*mm^2  BasedOnType=Density  Density=1000  DensityUnits=kg/m^3  DoExposeReferenceFrame=on  SerializedFrames=<Frames/>  GraphicType=FromGeometry  MarkerShape=Sphere  MarkerSize=10  GraphicVisPropType=SimpleVisualProperties  GraphicDiffuseColor=smiData.Solid(8).color  GraphicSpecularColor=[0.5 0.5 0.5 1.0]  GraphicAmbientColor=[0.15 0.15 0.15 1.0]  GraphicEmissiveColor=[0.0 0.0 0.0 1.0]  GraphicShininess=75  GraphicOpacity=smiData.Solid(8).opacity
  F : PMIOPort  Side=Left
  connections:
  ReferenceFrame/RConn1 -- Solid/RConn1 -- F/RConn1

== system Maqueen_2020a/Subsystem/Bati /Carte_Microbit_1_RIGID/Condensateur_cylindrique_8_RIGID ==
  ReferenceFrame : sm_lib/Frames and Transforms/Reference Frame
  Solid : sm_lib/Body Elements/File Solid  ExtGeomFileName=Condensateur cylindrique_Defaut_sldprt.STL  UnitType=Custom  ExtGeomFileUnits=mm  StepReaderType=HEX  ExportConvexHullGeometry=off  InertiaType=Custom  Mass=smiData.Solid(8).mass  MassUnits=kg  CenterOfMass=smiData.Solid(8).CoM  CenterOfMassUnits=mm  MomentsOfInertia=smiData.Solid(8).MoI  MomentsOfInertiaUnits=kg*mm^2  ProductsOfInertia=smiData.Solid(8).PoI  ProductsOfInertiaUnits=kg*mm^2  BasedOnType=Density  Density=1000  DensityUnits=kg/m^3  DoExposeReferenceFrame=on  SerializedFrames=<Frames/>  GraphicType=FromGeometry  MarkerShape=Sphere  MarkerSize=10  GraphicVisPropType=SimpleVisualProperties  GraphicDiffuseColor=smiData.Solid(8).color  GraphicSpecularColor=[0.5 0.5 0.5 1.0]  GraphicAmbientColor=[0.15 0.15 0.15 1.0]  GraphicEmissiveColor=[0.0 0.0 0.0 1.0]  GraphicShininess=75  GraphicOpacity=smiData.Solid(8).opacity
  F : PMIOPort  Side=Left
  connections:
  ReferenceFrame/RConn1 -- Solid/RConn1 -- F/RConn1

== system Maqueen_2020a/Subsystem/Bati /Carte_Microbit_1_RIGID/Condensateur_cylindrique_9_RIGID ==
  ReferenceFrame : sm_lib/Frames and Transforms/Reference Frame
  Solid : sm_lib/Body Elements/File Solid  ExtGeomFileName=Condensateur cylindrique_Defaut_sldprt.STL  UnitType=Custom  ExtGeomFileUnits=mm  StepReaderType=HEX  ExportConvexHullGeometry=off  InertiaType=Custom  Mass=smiData.Solid(8).mass  MassUnits=kg  CenterOfMass=smiData.Solid(8).CoM  CenterOfMassUnits=mm  MomentsOfInertia=smiData.Solid(8).MoI  MomentsOfInertiaUnits=kg*mm^2  ProductsOfInertia=smiData.Solid(8).PoI  ProductsOfInertiaUnits=kg*mm^2  BasedOnType=Density  Density=1000  DensityUnits=kg/m^3  DoExposeReferenceFrame=on  SerializedFrames=<Frames/>  GraphicType=FromGeometry  MarkerShape=Sphere  MarkerSize=10  GraphicVisPropType=SimpleVisualProperties  GraphicDiffuseColor=smiData.Solid(8).color  GraphicSpecularColor=[0.5 0.5 0.5 1.0]  GraphicAmbientColor=[0.15 0.15 0.15 1.0]  GraphicEmissiveColor=[0.0 0.0 0.0 1.0]  GraphicShininess=75  GraphicOpacity=smiData.Solid(8).opacity
  F : PMIOPort  Side=Left
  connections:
  ReferenceFrame/RConn1 -- Solid/RConn1 -- F/RConn1

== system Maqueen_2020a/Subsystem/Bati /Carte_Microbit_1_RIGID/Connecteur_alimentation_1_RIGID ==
  ReferenceFrame : sm_lib/Frames and Transforms/Reference Frame
  Solid : sm_lib/Body Elements/File Solid  ExtGeomFileName=Connecteur alimentation_Defaut_sldprt.STL  UnitType=Custom  ExtGeomFileUnits=mm  StepReaderType=HEX  ExportConvexHullGeometry=off  InertiaType=Custom  Mass=smiData.Solid(16).mass  MassUnits=kg  CenterOfMass=smiData.Solid(16).CoM  CenterOfMassUnits=mm  MomentsOfInertia=smiData.Solid(16).MoI  MomentsOfInertiaUnits=kg*mm^2  ProductsOfInertia=smiData.Solid(16).PoI  ProductsOfInertiaUnits=kg*mm^2  BasedOnType=Density  Density=1000  DensityUnits=kg/m^3  DoExposeReferenceFrame=on  SerializedFrames=<Frames/>  GraphicType=FromGeometry  MarkerShape=Sphere  MarkerSize=10  GraphicVisPropType=SimpleVisualProperties  GraphicDiffuseColor=smiData.Solid(16).color  GraphicSpecularColor=[0.5 0.5 0.5 1.0]  GraphicAmbientColor=[0.15 0.15 0.15 1.0]  GraphicEmissiveColor=[0.0 0.0 0.0 1.0]  GraphicShininess=75  GraphicOpacity=smiData.Solid(16).opacity
  F : PMIOPort  Side=Left
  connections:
  ReferenceFrame/RConn1 -- Solid/RConn1 -- F/RConn1

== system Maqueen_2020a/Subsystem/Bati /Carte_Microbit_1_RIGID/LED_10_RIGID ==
  ReferenceFrame : sm_lib/Frames and Transforms/Reference Frame
  Solid : sm_lib/Body Elements/File Solid  ExtGeomFileName=LED_Defaut_sldprt.STL  UnitType=Custom  ExtGeomFileUnits=mm  StepReaderType=HEX  ExportConvexHullGeometry=off  InertiaType=Custom  Mass=smiData.Solid(10).mass  MassUnits=kg  CenterOfMass=smiData.Solid(10).CoM  CenterOfMassUnits=mm  MomentsOfInertia=smiData.Solid(10).MoI  MomentsOfInertiaUnits=kg*mm^2  ProductsOfInertia=smiData.Solid(10).PoI  ProductsOfInertiaUnits=kg*mm^2  BasedOnType=Density  Density=1000  DensityUnits=kg/m^3  DoExposeReferenceFrame=on  SerializedFrames=<Frames/>  GraphicType=FromGeometry  MarkerShape=Sphere  MarkerSize=10  GraphicVisPropType=SimpleVisualProperties  GraphicDiffuseColor=smiData.Solid(10).color  GraphicSpecularColor=[0.5 0.5 0.5 1.0]  GraphicAmbientColor=[0.15 0.15 0.15 1.0]  GraphicEmissiveColor=[0.0 0.0 0.0 1.0]  GraphicShininess=75  GraphicOpacity=smiData.Solid(10).opacity
  F : PMIOPort  Side=Left
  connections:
  ReferenceFrame/RConn1 -- Solid/RConn1 -- F/RConn1

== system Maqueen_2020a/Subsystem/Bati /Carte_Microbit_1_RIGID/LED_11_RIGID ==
  ReferenceFrame : sm_lib/Frames and Transforms/Reference Frame
  Solid : sm_lib/Body Elements/File Solid  ExtGeomFileName=LED_Defaut_sldprt.STL  UnitType=Custom  ExtGeomFileUnits=mm  StepReaderType=HEX  ExportConvexHullGeometry=off  InertiaType=Custom  Mass=smiData.Solid(10).mass  MassUnits=kg  CenterOfMass=smiData.Solid(10).CoM  CenterOfMassUnits=mm  MomentsOfInertia=smiData.Solid(10).MoI  MomentsOfInertiaUnits=kg*mm^2  ProductsOfInertia=smiData.Solid(10).PoI  ProductsOfInertiaUnits=kg*mm^2  BasedOnType=Density  Density=1000  DensityUnits=kg/m^3  DoExposeReferenceFrame=on  SerializedFrames=<Frames/>  GraphicType=FromGeometry  MarkerShape=Sphere  MarkerSize=10  GraphicVisPropType=SimpleVisualProperties  GraphicDiffuseColor=smiData.Solid(10).color  GraphicSpecularColor=[0.5 0.5 0.5 1.0]  GraphicAmbientColor=[0.15 0.15 0.15 1.0]  GraphicEmissiveColor=[0.0 0.0 0.0 1.0]  GraphicShininess=75  GraphicOpacity=smiData.Solid(10).opacity
  F : PMIOPort  Side=Left
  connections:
  ReferenceFrame/RConn1 -- Solid/RConn1 -- F/RConn1

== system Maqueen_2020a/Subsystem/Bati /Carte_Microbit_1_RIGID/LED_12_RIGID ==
  ReferenceFrame : sm_lib/Frames and Transforms/Reference Frame
  Solid : sm_lib/Body Elements/File Solid  ExtGeomFileName=LED_Defaut_sldprt.STL  UnitType=Custom  ExtGeomFileUnits=mm  StepReaderType=HEX  ExportConvexHullGeometry=off  InertiaType=Custom  Mass=smiData.Solid(10).mass  MassUnits=kg  CenterOfMass=smiData.Solid(10).CoM  CenterOfMassUnits=mm  MomentsOfInertia=smiData.Solid(10).MoI  MomentsOfInertiaUnits=kg*mm^2  ProductsOfInertia=smiData.Solid(10).PoI  ProductsOfInertiaUnits=kg*mm^2  BasedOnType=Density  Density=1000  DensityUnits=kg/m^3  DoExposeReferenceFrame=on  SerializedFrames=<Frames/>  GraphicType=FromGeometry  MarkerShape=Sphere  MarkerSize=10  GraphicVisPropType=SimpleVisualProperties  GraphicDiffuseColor=smiData.Solid(10).color  GraphicSpecularColor=[0.5 0.5 0.5 1.0]  GraphicAmbientColor=[0.15 0.15 0.15 1.0]  GraphicEmissiveColor=[0.0 0.0 0.0 1.0]  GraphicShininess=75  GraphicOpacity=smiData.Solid(10).opacity
  F : PMIOPort  Side=Left
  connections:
  ReferenceFrame/RConn1 -- Solid/RConn1 -- F/RConn1

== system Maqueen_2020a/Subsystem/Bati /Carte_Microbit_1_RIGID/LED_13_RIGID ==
  ReferenceFrame : sm_lib/Frames and Transforms/Reference Frame
  Solid : sm_lib/Body Elements/File Solid  ExtGeomFileName=LED_Defaut_sldprt.STL  UnitType=Custom  ExtGeomFileUnits=mm  StepReaderType=HEX  ExportConvexHullGeometry=off  InertiaType=Custom  Mass=smiData.Solid(10).mass  MassUnits=kg  CenterOfMass=smiData.Solid(10).CoM  CenterOfMassUnits=mm  MomentsOfInertia=smiData.Solid(10).MoI  MomentsOfInertiaUnits=kg*mm^2  ProductsOfInertia=smiData.Solid(10).PoI  ProductsOfInertiaUnits=kg*mm^2  BasedOnType=Density  Density=1000  DensityUnits=kg/m^3  DoExposeReferenceFrame=on  SerializedFrames=<Frames/>  GraphicType=FromGeometry  MarkerShape=Sphere  MarkerSize=10  GraphicVisPropType=SimpleVisualProperties  GraphicDiffuseColor=smiData.Solid(10).color  GraphicSpecularColor=[0.5 0.5 0.5 1.0]  GraphicAmbientColor=[0.15 0.15 0.15 1.0]  GraphicEmissiveColor=[0.0 0.0 0.0 1.0]  GraphicShininess=75  GraphicOpacity=smiData.Solid(10).opacity
  F : PMIOPort  Side=Left
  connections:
  ReferenceFrame/RConn1 -- Solid/RConn1 -- F/RConn1

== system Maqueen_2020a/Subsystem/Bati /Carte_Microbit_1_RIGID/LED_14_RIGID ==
  ReferenceFrame : sm_lib/Frames and Transforms/Reference Frame
  Solid : sm_lib/Body Elements/File Solid  ExtGeomFileName=LED_Defaut_sldprt.STL  UnitType=Custom  ExtGeomFileUnits=mm  StepReaderType=HEX  ExportConvexHullGeometry=off  InertiaType=Custom  Mass=smiData.Solid(10).mass  MassUnits=kg  CenterOfMass=smiData.Solid(10).CoM  CenterOfMassUnits=mm  MomentsOfInertia=smiData.Solid(10).MoI  MomentsOfInertiaUnits=kg*mm^2  ProductsOfInertia=smiData.Solid(10).PoI  ProductsOfInertiaUnits=kg*mm^2  BasedOnType=Density  Density=1000  DensityUnits=kg/m^3  DoExposeReferenceFrame=on  SerializedFrames=<Frames/>  GraphicType=FromGeometry  MarkerShape=Sphere  MarkerSize=10  GraphicVisPropType=SimpleVisualProperties  GraphicDiffuseColor=smiData.Solid(10).color  GraphicSpecularColor=[0.5 0.5 0.5 1.0]  GraphicAmbientColor=[0.15 0.15 0.15 1.0]  GraphicEmissiveColor=[0.0 0.0 0.0 1.0]  GraphicShininess=75  GraphicOpacity=smiData.Solid(10).opacity
  F : PMIOPort  Side=Left
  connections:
  ReferenceFrame/RConn1 -- Solid/RConn1 -- F/RConn1

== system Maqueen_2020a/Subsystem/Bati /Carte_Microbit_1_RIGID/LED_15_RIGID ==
  ReferenceFrame : sm_lib/Frames and Transforms/Reference Frame
  Solid : sm_lib/Body Elements/File Solid  ExtGeomFileName=LED_Defaut_sldprt.STL  UnitType=Custom  ExtGeomFileUnits=mm  StepReaderType=HEX  ExportConvexHullGeometry=off  InertiaType=Custom  Mass=smiData.Solid(10).mass  MassUnits=kg  CenterOfMass=smiData.Solid(10).CoM  CenterOfMassUnits=mm  MomentsOfInertia=smiData.Solid(10).MoI  MomentsOfInertiaUnits=kg*mm^2  ProductsOfInertia=smiData.Solid(10).PoI  ProductsOfInertiaUnits=kg*mm^2  BasedOnType=Density  Density=1000  DensityUnits=kg/m^3  DoExposeReferenceFrame=on  SerializedFrames=<Frames/>  GraphicType=FromGeometry  MarkerShape=Sphere  MarkerSize=10  GraphicVisPropType=SimpleVisualProperties  GraphicDiffuseColor=smiData.Solid(10).color  GraphicSpecularColor=[0.5 0.5 0.5 1.0]  GraphicAmbientColor=[0.15 0.15 0.15 1.0]  GraphicEmissiveColor=[0.0 0.0 0.0 1.0]  GraphicShininess=75  GraphicOpacity=smiData.Solid(10).opacity
  F : PMIOPort  Side=Left
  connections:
  ReferenceFrame/RConn1 -- Solid/RConn1 -- F/RConn1

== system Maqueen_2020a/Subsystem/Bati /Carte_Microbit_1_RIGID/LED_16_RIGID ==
  ReferenceFrame : sm_lib/Frames and Transforms/Reference Frame
  Solid : sm_lib/Body Elements/File Solid  ExtGeomFileName=LED_Defaut_sldprt.STL  UnitType=Custom  ExtGeomFileUnits=mm  StepReaderType=HEX  ExportConvexHullGeometry=off  InertiaType=Custom  Mass=smiData.Solid(10).mass  MassUnits=kg  CenterOfMass=smiData.Solid(10).CoM  CenterOfMassUnits=mm  MomentsOfInertia=smiData.Solid(10).MoI  MomentsOfInertiaUnits=kg*mm^2  ProductsOfInertia=smiData.Solid(10).PoI  ProductsOfInertiaUnits=kg*mm^2  BasedOnType=Density  Density=1000  DensityUnits=kg/m^3  DoExposeReferenceFrame=on  SerializedFrames=<Frames/>  GraphicType=FromGeometry  MarkerShape=Sphere  MarkerSize=10  GraphicVisPropType=SimpleVisualProperties  GraphicDiffuseColor=smiData.Solid(10).color  GraphicSpecularColor=[0.5 0.5 0.5 1.0]  GraphicAmbientColor=[0.15 0.15 0.15 1.0]  GraphicEmissiveColor=[0.0 0.0 0.0 1.0]  GraphicShininess=75  GraphicOpacity=smiData.Solid(10).opacity
  F : PMIOPort  Side=Left
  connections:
  ReferenceFrame/RConn1 -- Solid/RConn1 -- F/RConn1

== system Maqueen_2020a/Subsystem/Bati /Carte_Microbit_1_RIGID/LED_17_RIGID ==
  ReferenceFrame : sm_lib/Frames and Transforms/Reference Frame
  Solid : sm_lib/Body Elements/File Solid  ExtGeomFileName=LED_Defaut_sldprt.STL  UnitType=Custom  ExtGeomFileUnits=mm  StepReaderType=HEX  ExportConvexHullGeometry=off  InertiaType=Custom  Mass=smiData.Solid(10).mass  MassUnits=kg  CenterOfMass=smiData.Solid(10).CoM  CenterOfMassUnits=mm  MomentsOfInertia=smiData.Solid(10).MoI  MomentsOfInertiaUnits=kg*mm^2  ProductsOfInertia=smiData.Solid(10).PoI  ProductsOfInertiaUnits=kg*mm^2  BasedOnType=Density  Density=1000  DensityUnits=kg/m^3  DoExposeReferenceFrame=on  SerializedFrames=<Frames/>  GraphicType=FromGeometry  MarkerShape=Sphere  MarkerSize=10  GraphicVisPropType=SimpleVisualProperties  GraphicDiffuseColor=smiData.Solid(10).color  GraphicSpecularColor=[0.5 0.5 0.5 1.0]  GraphicAmbientColor=[0.15 0.15 0.15 1.0]  GraphicEmissiveColor=[0.0 0.0 0.0 1.0]  GraphicShininess=75  GraphicOpacity=smiData.Solid(10).opacity
  F : PMIOPort  Side=Left
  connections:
  ReferenceFrame/RConn1 -- Solid/RConn1 -- F/RConn1

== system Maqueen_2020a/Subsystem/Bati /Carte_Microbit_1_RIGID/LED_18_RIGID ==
  ReferenceFrame : sm_lib/Frames and Transforms/Reference Frame
  Solid : sm_lib/Body Elements/File Solid  ExtGeomFileName=LED_Defaut_sldprt.STL  UnitType=Custom  ExtGeomFileUnits=mm  StepReaderType=HEX  ExportConvexHullGeometry=off  InertiaType=Custom  Mass=smiData.Solid(10).mass  MassUnits=kg  CenterOfMass=smiData.Solid(10).CoM  CenterOfMassUnits=mm  MomentsOfInertia=smiData.Solid(10).MoI  MomentsOfInertiaUnits=kg*mm^2  ProductsOfInertia=smiData.Solid(10).PoI  ProductsOfInertiaUnits=kg*mm^2  BasedOnType=Density  Density=1000  DensityUnits=kg/m^3  DoExposeReferenceFrame=on  SerializedFrames=<Frames/>  GraphicType=FromGeometry  MarkerShape=Sphere  MarkerSize=10  GraphicVisPropType=SimpleVisualProperties  GraphicDiffuseColor=smiData.Solid(10).color  GraphicSpecularColor=[0.5 0.5 0.5 1.0]  GraphicAmbientColor=[0.15 0.15 0.15 1.0]  GraphicEmissiveColor=[0.0 0.0 0.0 1.0]  GraphicShininess=75  GraphicOpacity=smiData.Solid(10).opacity
  F : PMIOPort  Side=Left
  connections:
  ReferenceFrame/RConn1 -- Solid/RConn1 -- F/RConn1

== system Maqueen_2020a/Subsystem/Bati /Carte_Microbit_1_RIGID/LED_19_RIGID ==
  ReferenceFrame : sm_lib/Frames and Transforms/Reference Frame
  Solid : sm_lib/Body Elements/File Solid  ExtGeomFileName=LED_Defaut_sldprt.STL  UnitType=Custom  ExtGeomFileUnits=mm  StepReaderType=HEX  ExportConvexHullGeometry=off  InertiaType=Custom  Mass=smiData.Solid(10).mass  MassUnits=kg  CenterOfMass=smiData.Solid(10).CoM  CenterOfMassUnits=mm  MomentsOfInertia=smiData.Solid(10).MoI  MomentsOfInertiaUnits=kg*mm^2  ProductsOfInertia=smiData.Solid(10).PoI  ProductsOfInertiaUnits=kg*mm^2  BasedOnType=Density  Density=1000  DensityUnits=kg/m^3  DoExposeReferenceFrame=on  SerializedFrames=<Frames/>  GraphicType=FromGeometry  MarkerShape=Sphere  MarkerSize=10  GraphicVisPropType=SimpleVisualProperties  GraphicDiffuseColor=smiData.Solid(10).color  GraphicSpecularColor=[0.5 0.5 0.5 1.0]  GraphicAmbientColor=[0.15 0.15 0.15 1.0]  GraphicEmissiveColor=[0.0 0.0 0.0 1.0]  GraphicShininess=75  GraphicOpacity=smiData.Solid(10).opacity
  F : PMIOPort  Side=Left
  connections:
  ReferenceFrame/RConn1 -- Solid/RConn1 -- F/RConn1
